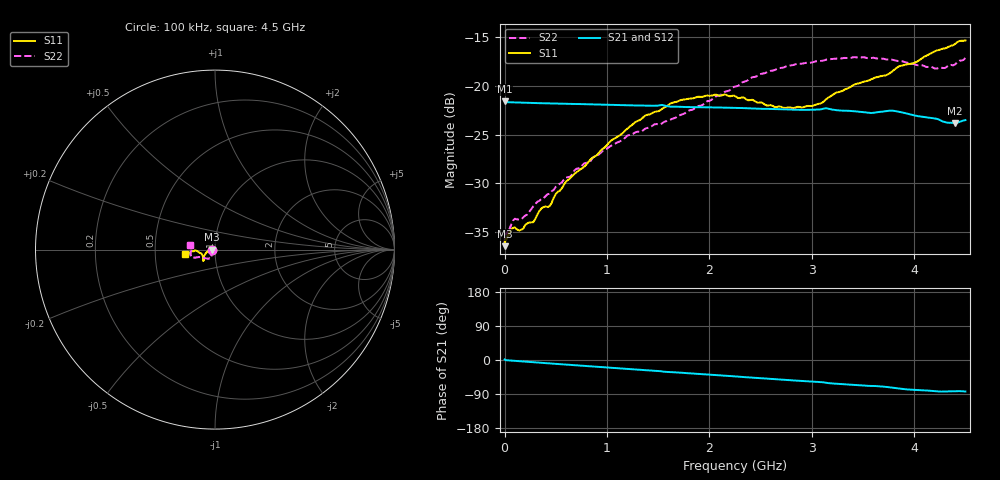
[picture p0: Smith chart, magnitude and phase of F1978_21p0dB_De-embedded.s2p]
! Integrated Device Technology
! Corporate Headquarters
! 6024 Silver Creek Valley Road
! San Jose, CA 95138  USA
! Phone:  1-408-284-8200
! Toll Free:  1-800-223-1366
! Webpage:  http://www.idt.com/
! Timing and RF Division
! 515 Groton Road, Suite 102
! Westford, MA 01886-6024
! Device:  F1978
! Description: 6-bit, 75 ohm, 0.5 dB Digital Step Attenuator
! Frequency:  5.0 MHz -  3.00 GHz
! Package:  4x4 mm QFN Plastic Package: 20 pin
! Ports:  2 RF, 11 DC
!  Pin  1  = D5 (16 dB)
!  Pin  2  = RF1  =  Port 1
!  Pin  3  = Serial Data In (DATA)
!  Pin  4  = Serial Clock (CLK)
!  Pin  5  = Serial Latch Enable (LE)
!  Pin  6  = VDD
!  Pin  7  = NC
!  Pin  8  = NC
!  Pin  9  = NC
!  Pin 10  = GND
!  Pin 11  = GND
!  Pin 12  = NC
!  Pin 13  = VMODE
!  Pin 14  = RF2  =  Port 2
!  Pin 15  = D4 (8 dB)
!  Pin 16  = D3 (4 dB)
!  Pin 17  = D2 (2 dB)
!  Pin 18  = NC
!  Pin 19  = D1 (1 dB)
!  Pin 20  = D0 (0.5 dB)
! State:  42
! Atten State:  21.0 dB
! Voltage:  +3.30 Volts
! Current:  0.592 mA
! Data:  The device was measured on a F1975 evaluation board which has
!  individual transmission lines to the RF pins.  Data was collected
!  using a calibrated network analyzer.  The evaluation board was
!  de-embedded using Automatic Fixture Removal (AFR).
!  The reference plane is the edge of the package pin.
! Misc:
!  Action Tracker AT0416
! Date Measured:  2018-02-08
! Date:  2018-03-26  MJV
! Note:
!  Integrated Device Technology supplies this data as a sample of measured
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# GHz S dB R 75
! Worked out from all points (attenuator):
!   291 points, 100 kHz to 4.5 GHz, reference 75 ohm
!   highest |S21| = -21.59 dB at 100 kHz (marker M1); lowest = -23.8 dB at 4.4 GHz (marker M2)
!   lowest |S11| = -36.5 dB at 100 kHz (marker M3), VSWR 1.03, Z = 72.8 - j0.00879 ohm
!   |S11| at or under -10 dB: start of sweep to end of sweep
!   |S22| runs from -36.3 to -17.0 dB; largest |S21 - S12| = 0.00014
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0.0001  -36.47 -179.8  -21.59 1.2  -21.58 1.3  -36.32 -178.2
0.003  -36.00 -178.3  -21.63 0.7  -21.62 0.7  -35.63 -177.2
0.01  -35.85 -178.2  -21.66 -0.4  -21.65 -0.4  -35.33 -175.0
0.1  -34.55 -175.1  -21.69 -2.3  -21.69 -2.3  -33.65 -159.0
0.16  -34.80 -177.3  -21.72 -3.5  -21.71 -3.5  -33.73 -150.5
0.28  -34.01 -180.0  -21.75 -5.9  -21.75 -5.9  -32.37 -140.6
0.36  -32.59 179.9  -21.77 -7.5  -21.77 -7.5  -31.59 -132.7
0.44  -32.37 -179.4  -21.79 -9.0  -21.79 -9.0  -31.09 -127.2
0.6  -29.82 -175.6  -21.83 -12.1  -21.83 -12.1  -29.42 -122.7
0.76  -28.44 -168.7  -21.87 -15.2  -21.87 -15.2  -28.14 -120.6
1.28  -23.70 -152.4  -22.00 -25.1  -22.00 -25.1  -24.75 -121.5
1.52  -22.51 -145.3  -21.98 -29.5  -21.97 -29.5  -23.94 -128.4
1.64  -21.72 -142.5  -22.13 -32.2  -22.13 -32.1  -23.36 -132.4
1.88  -21.12 -138.5  -22.18 -36.4  -22.18 -36.3  -22.10 -143.5
2.26  -21.10 -137.0  -22.25 -43.5  -22.25 -43.5  -20.04 -154.8
2.64  -22.18 -147.4  -22.37 -50.6  -22.37 -50.6  -18.35 -158.3
3.02  -21.99 -164.1  -22.44 -57.3  -22.43 -57.3  -17.52 -161.1
3.42  -19.84 -175.6  -22.61 -66.1  -22.61 -66.1  -17.03 -166.9
3.76  -18.70 -175.7  -22.54 -72.1  -22.53 -72.1  -17.29 -173.6
4.2  -16.44 -172.6  -23.34 -82.0  -23.33 -82.0  -18.20 174.5
4.4  -15.67 -170.2  -23.81 -82.5  -23.80 -82.5  -17.79 171.1
4.5  -15.32 -171.9  -23.51 -83.3  -23.50 -83.3  -17.12 169.7
